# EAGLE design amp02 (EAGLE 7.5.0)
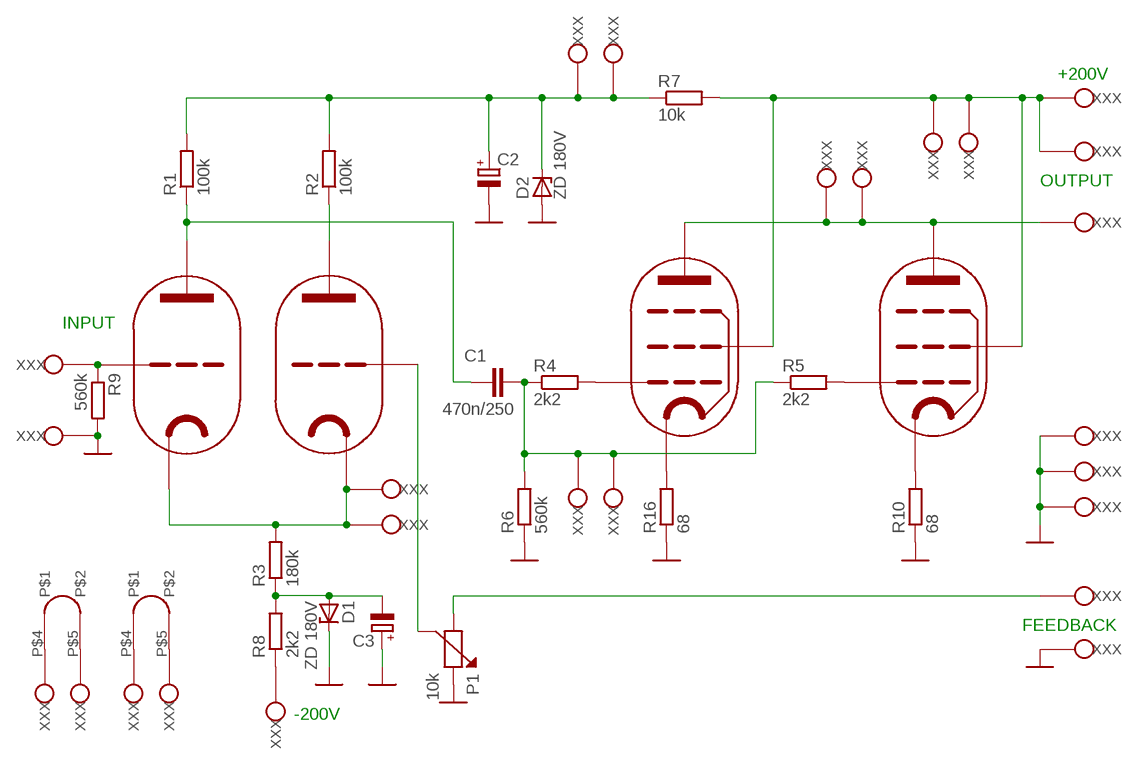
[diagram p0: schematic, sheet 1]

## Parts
C1  470n/250  C-EU150-072X183  [C150-072X183]
C2  CPOL-EUE5-13  [E5-13]
C3  CPOL-EUE5-13  [E5-13]
D1  ZD 180V  BZD23  [SOD81]
D2  ZD 180V  BZD23  [SOD81]
INPUT  PIN  [PIN]
OUTPUT  PIN  [PIN]
OUTPUT1  PIN  [PIN]
OUTPUT2  PIN  [PIN]
OUTPUT3  PIN  [PIN]
OUTPUT4  PIN  [PIN]
P1  10k  P10V  [PT10V]
R1  100k  R-EU_0207/10  [0207/10]
R2  100k  R-EU_0207/10  [0207/10]
R3  180k  R-EU_0207/10  [0207/10]
R4  2k2  R-EU_0207/10  [0207/10]
R5  2k2  R-EU_0207/10  [0207/10]
R6  560k  R-EU_0207/10  [0207/10]
R7  10k  R-EU_0207/10  [0207/10]
R8  2k2  R-EU_0207/10  [0207/10]
R9  560k  R-EU_0207/10  [0207/10]
R10  68  R-EU_0207/10  [0207/10]
R16  68  R-EU_0207/10  [0207/10]
U$1  PCL86  [NOVAL02]
U$2  PCL86  [NOVAL02]
U$3  PIN  [PIN]
U$4  PIN  [PIN]
U$5  PIN  [PIN]
U$6  PIN  [PIN]
U$7  PIN  [PIN]
U$8  PIN  [PIN]
U$9  PIN  [PIN]
U$10  PIN  [PIN]
U$11  PIN  [PIN]
U$12  PIN  [PIN]
U$13  PIN  [PIN]
U$14  PIN  [PIN]
U$15  PIN  [PIN]
U$16  PIN  [PIN]
U$17  PIN  [PIN]
U$18  PIN  [PIN]
U$19  PIN  [PIN]
U$20  PIN  [PIN]
U$21  PIN  [PIN]

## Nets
GND: C2.- C3.+ D1.C D2.A OUTPUT4.P$1(XXX) P1.2(K) R6.1 R9.2 R10.1 R16.1 U$10.P$1(XXX) U$16.P$1(XXX) U$17.P$1(XXX) U$19.P$1(XXX)
N$1: C1.1 R1.1 U$1.P$9(A)
N$2: R2.1 U$2.P$9(A)
N$3: R3.2 U$1.P$2(K) U$2.P$2(K) U$5.P$1(XXX) U$6.P$1(XXX)
N$4: OUTPUT1.P$1(XXX) OUTPUT2.P$1(XXX) R7.2 U$1.P$3(G2) U$2.P$3(G2) U$13.P$1(XXX) U$18.P$1(XXX)
N$5: OUTPUT.P$1(XXX) U$1.P$6(A) U$2.P$6(A) U$9.P$1(XXX) U$12.P$1(XXX)
N$6: C1.2 R4.1 R5.1 R6.2 U$7.P$1(XXX) U$8.P$1(XXX)
N$7: P1.3(J) U$2.P$1(G1)
N$8: R4.2 U$1.P$8(G1)
N$9: R5.2 U$2.P$8(G1)
N$10: U$1.P$5 U$3.P$1(XXX)
N$11: U$2.P$4 U$4.P$1(XXX)
N$12: U$1.P$4 U$14.P$1(XXX)
N$13: INPUT.P$1(XXX) R9.1 U$1.P$1(G1)
N$14: R10.2 U$2.P$7(K)
N$15: R16.2 U$1.P$7(K)
N$16: C2.+ D2.C R1.2 R2.2 R7.1 U$20.P$1(XXX) U$21.P$1(XXX)
N$17: R8.1 U$11.P$1(XXX)
N$18: C3.- D1.A R3.1 R8.2
N$20: OUTPUT3.P$1(XXX) P1.1(Z)
N$23: U$2.P$5 U$15.P$1(XXX)

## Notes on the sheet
- +200V
- OUTPUT
- INPUT
- FEEDBACK
- -200V

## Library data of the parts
C1 = rcl:C-EU: CAPACITOR, European symbol
C2 C3 = rcl:CPOL-EU: POLARIZED CAPACITOR, European symbol
D1 D2 = diode:BZD23: Z DIODE
INPUT OUTPUT OUTPUT1-OUTPUT4 U$3-U$21 = lampy03:PIN
P1 = lampy02:P10V
R1-R10 R16 = rcl:R-EU_: RESISTOR, European symbol
U$1 U$2 = lampy03:PCL86

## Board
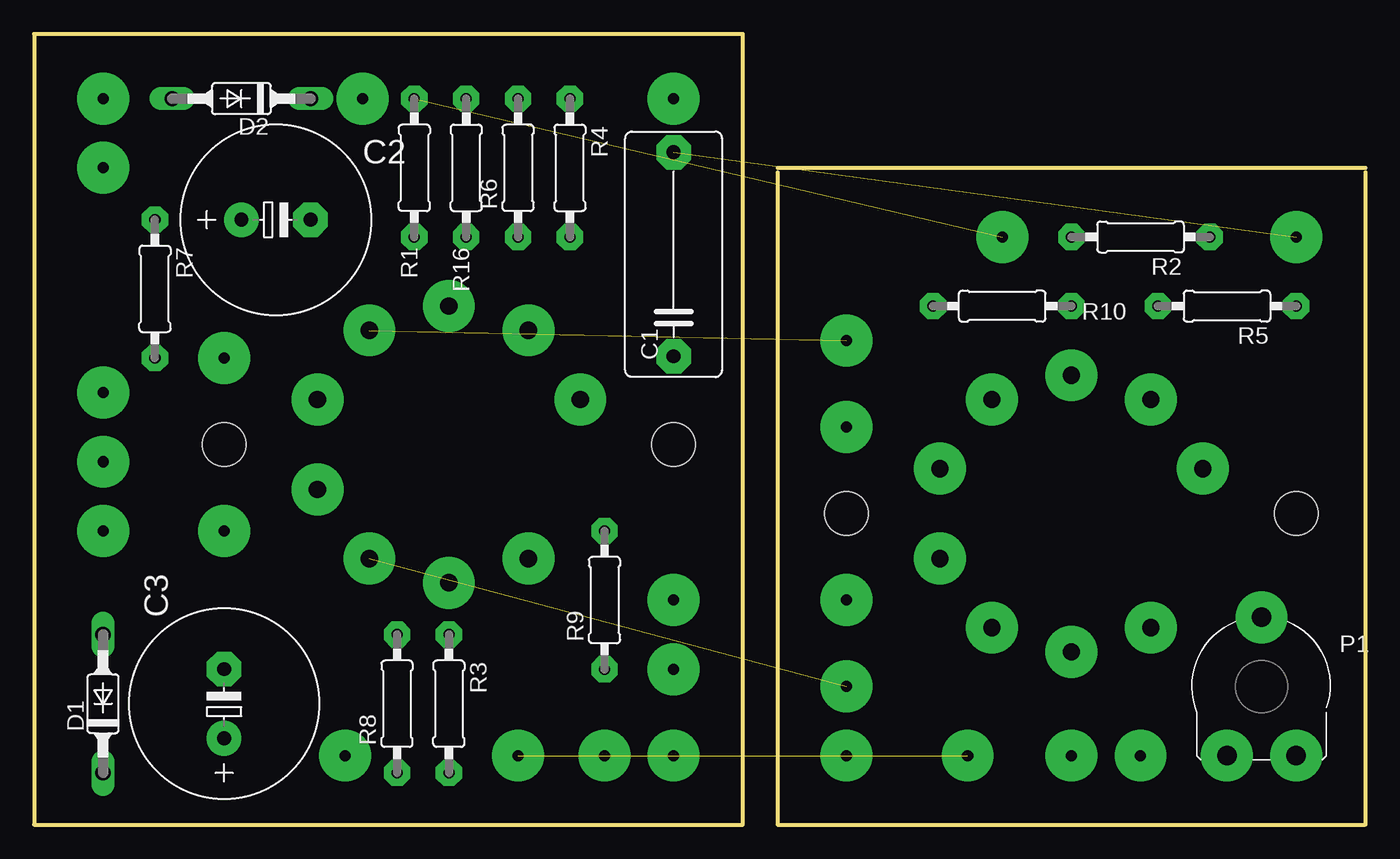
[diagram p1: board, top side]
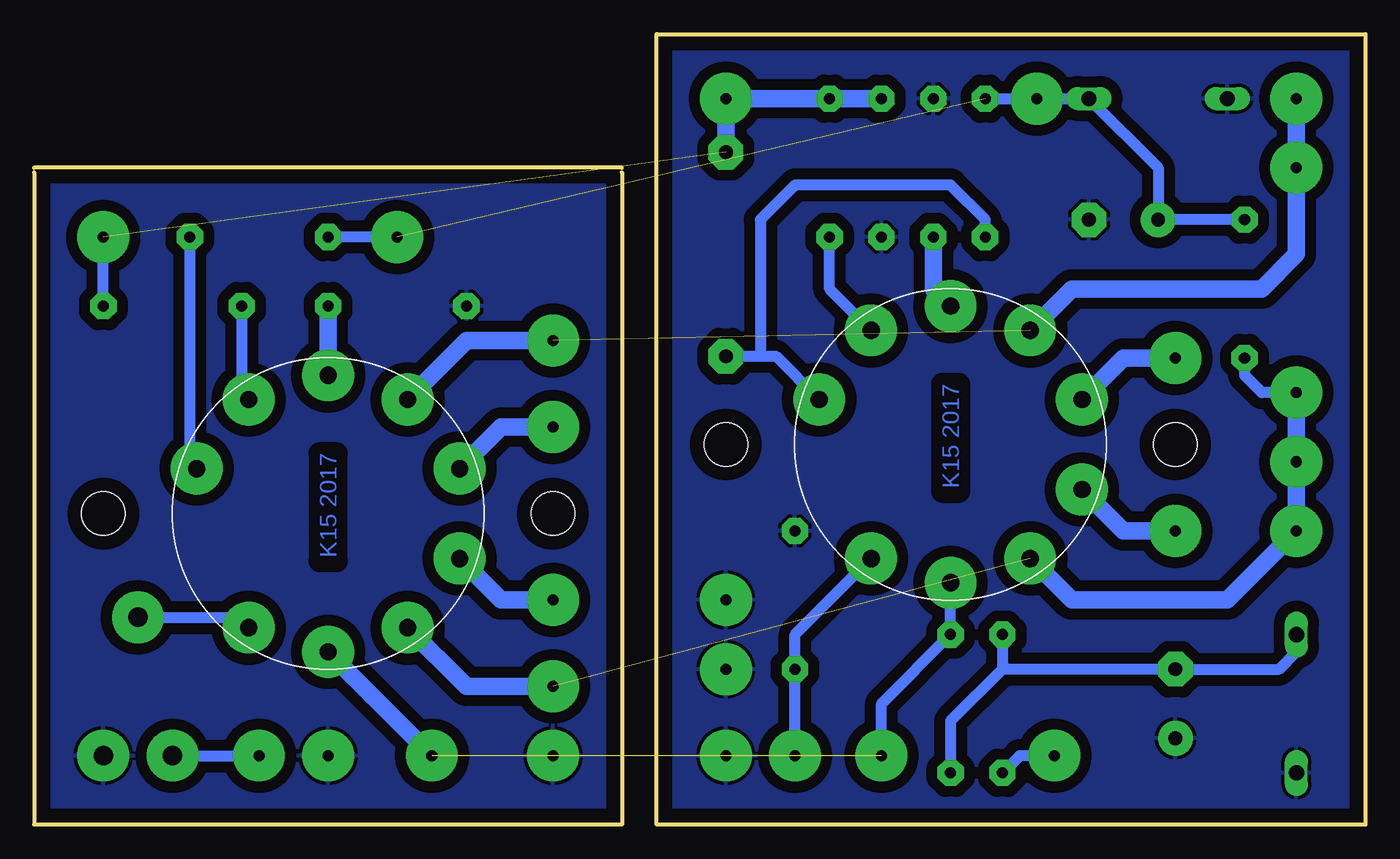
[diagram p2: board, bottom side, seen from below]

Size 97.79 x 58.09 mm. Coordinates in mm from the lower left corner, seen from the top.
Outline: 54.61,48.26 97.78,48.26
Outline: 54.61,47.93 54.61,0 97.79,0 97.79,47.93
Outline: 52.06,0 52.06,58.09 0,58.09 0,0 52.06,0
Copper layers (1*16): Top 0.035mm / dielectric 1.5mm / Bottom 0.035mm
Design rules "default": minimum track width 10mil, minimum drill 24mil, track to track 8mil, track to pad 8mil, pad to pad 8mil, via to via 8mil, smd to smd 8mil, copper to edge 40mil, drill to drill 8mil, minimum pad ring 10mil, minimum via ring 8mil, stop-mask expansion 4mil, vias tented up to drill 0mil, thermal gap 10mil
Holes 3.2 mm at 92.7,22.86 46.98,27.94 59.68,22.86 13.96,27.94

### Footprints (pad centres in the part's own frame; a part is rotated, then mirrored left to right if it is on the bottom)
C150-072X183 = drill 1.016 pad 2.54 octagon: 1 -7.493,0; 2 7.493,0
E5-13 = drill 1.016 pad 2.54: + -2.54,0 | drill 1.016 pad 2.54 octagon: - 2.54,0
SOD81 = drill 1.118 long: A 5.08,0; C -5.08,0
PIN = drill 0.813 pad 3.81: P$1 0,0
PT10V = drill 1.422 pad 3.81: 1 -2.54,-5.08; 2 2.54,-5.08; 3 0,5.08
0207/10 = drill 0.813 pad 1.93 octagon: 1 -5.08,0; 2 5.08,0
NOVAL02 = drill 1.27 pad 3.81: P$1 8.382,-5.842; P$2 10.16,0; P$3 8.382,5.842; P$4 3.302,9.652; P$5 -3.302,9.652; P$6 -8.382,5.842; P$7 -10.16,0; P$8 -8.382,-5.842; P$9 -3.302,-9.652

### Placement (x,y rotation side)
C1  46.98,41.91 90 top
C2  17.77,44.45 0 top
C3  13.96,8.89 90 top
D1  5.07,8.89 90 top
D2  15.23,53.34 180 top
INPUT  41.9,5.08 90 top
OUTPUT  5.07,48.26 90 top
OUTPUT1  5.07,21.59 90 top
OUTPUT2  5.07,26.67 90 top
OUTPUT3  81.27,5.08 90 top
OUTPUT4  46.98,5.08 90 top
P1  90.16,10.16 0 top
R1  27.93,48.26 90 top
R2  81.27,43.18 180 top
R3  30.47,8.89 90 top
R4  39.36,48.26 270 top
R5  87.62,38.1 180 top
R6  35.55,48.26 90 top
R7  8.88,39.37 270 top
R8  26.66,8.89 90 top
R9  41.9,16.51 90 top
R10  71.11,38.1 0 top
R16  31.74,48.26 270 top
U$1  30.47,27.94 270 bottom
U$2  76.19,22.86 270 bottom
U$3  13.96,34.29 90 top
U$4  59.68,16.51 90 top
U$5  35.55,5.08 90 top
U$6  68.57,5.08 90 top
U$7  46.98,53.34 90 top
U$8  92.7,43.18 90 top
U$9  5.07,53.34 90 top
U$10  46.98,11.43 90 top
U$11  22.85,5.08 90 top
U$12  59.68,35.56 90 top
U$13  5.07,31.75 90 top
U$14  13.96,21.59 90 top
U$15  59.68,29.21 90 top
U$16  46.98,16.51 90 top
U$17  76.19,5.08 90 top
U$18  59.68,10.16 90 top
U$19  59.68,5.08 90 top
U$20  24.12,53.34 90 top
U$21  71.11,43.18 90 top

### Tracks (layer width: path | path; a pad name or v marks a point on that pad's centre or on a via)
GND  (1 unrouted)
  pour Bottom (isolate 0.813): -0.01,0 -0.01,60.96 52.06,60.96 52.06,0
  pour Bottom (isolate 0.813): 54.6,0 54.6,48.26 97.78,48.26 97.78,0
N$1
  Bottom 0.813: C1.1 44.44,34.42 | 44.44,34.42 43.3,34.42 U$1.P$9 | R1.1 27.93,44.45 30.47,46.99 41.9,46.99 44.44,44.45 44.44,34.42
N$2
  Bottom 0.813: R2.1 86.35,26.67 U$2.P$9
N$3  (1 unrouted)
  Bottom 0.813: U$5.P$1 35.55,8.89 R3.2 U$1.P$2
  Bottom 1.27: U$2.P$2 U$6.P$1
N$4  (1 unrouted)
  Bottom 0.813: U$13.P$1 7.61,31.75 8.88,33.02 R7.2
  Bottom 1.27: U$13.P$1 OUTPUT2.P$1 OUTPUT1.P$1 10.15,16.51 21.58,16.51 U$1.P$3 | U$18.P$1 66.03,10.16 U$2.P$3
N$5  (1 unrouted)
  Bottom 1.27: U$9.P$1 OUTPUT.P$1 5.07,41.91 7.61,39.37 21.58,39.37 U$1.P$6 | U$12.P$1 66.03,35.56 U$2.P$6
N$6  (1 unrouted)
  Bottom 0.813: R5.1 U$8.P$1
  Bottom 1.27: C1.2 U$7.P$1 R6.2 R4.1
N$7
  Bottom 0.813: P1.3 82.79,15.24 U$2.P$1
N$8
  Bottom 0.813: U$1.P$8 39.36,39.37 R4.2
N$9
  Bottom 0.813: R5.2 82.54,31.75 U$2.P$8
N$10
  Bottom 1.27: U$3.P$1 17.77,34.29 U$1.P$5
N$11
  Bottom 1.27: U$4.P$1 63.49,16.51 U$2.P$4
N$12
  Bottom 1.27: U$14.P$1 17.77,21.59 U$1.P$4
N$13
  Bottom 0.813: INPUT.P$1 R9.1 41.9,13.97 U$1.P$1
N$14
  Bottom 1.27: U$2.P$7 R10.2
N$15
  Bottom 1.27: R16.2 31.74,39.37 U$1.P$7
N$16  (1 unrouted)
  Bottom 0.813: R7.1 C2.+ 15.23,48.26 D2.C U$20.P$1 25.39,53.34 R1.2 | U$21.P$1 R2.2
N$17
  Bottom 0.813: U$11.P$1 25.39,5.08 R8.1
N$18
  Bottom 0.813: R8.2 26.66,11.43 | 26.66,11.43 30.47,7.62 R3.1 | D1.A 5.07,12.7 6.34,11.43 C3.- 26.66,11.43
N$20
  Bottom 0.813: P1.1 OUTPUT3.P$1
N$23
  Bottom 1.27: U$15.P$1 63.49,29.21 U$2.P$5

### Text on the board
Bottom: K15 2017 | K15 2017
